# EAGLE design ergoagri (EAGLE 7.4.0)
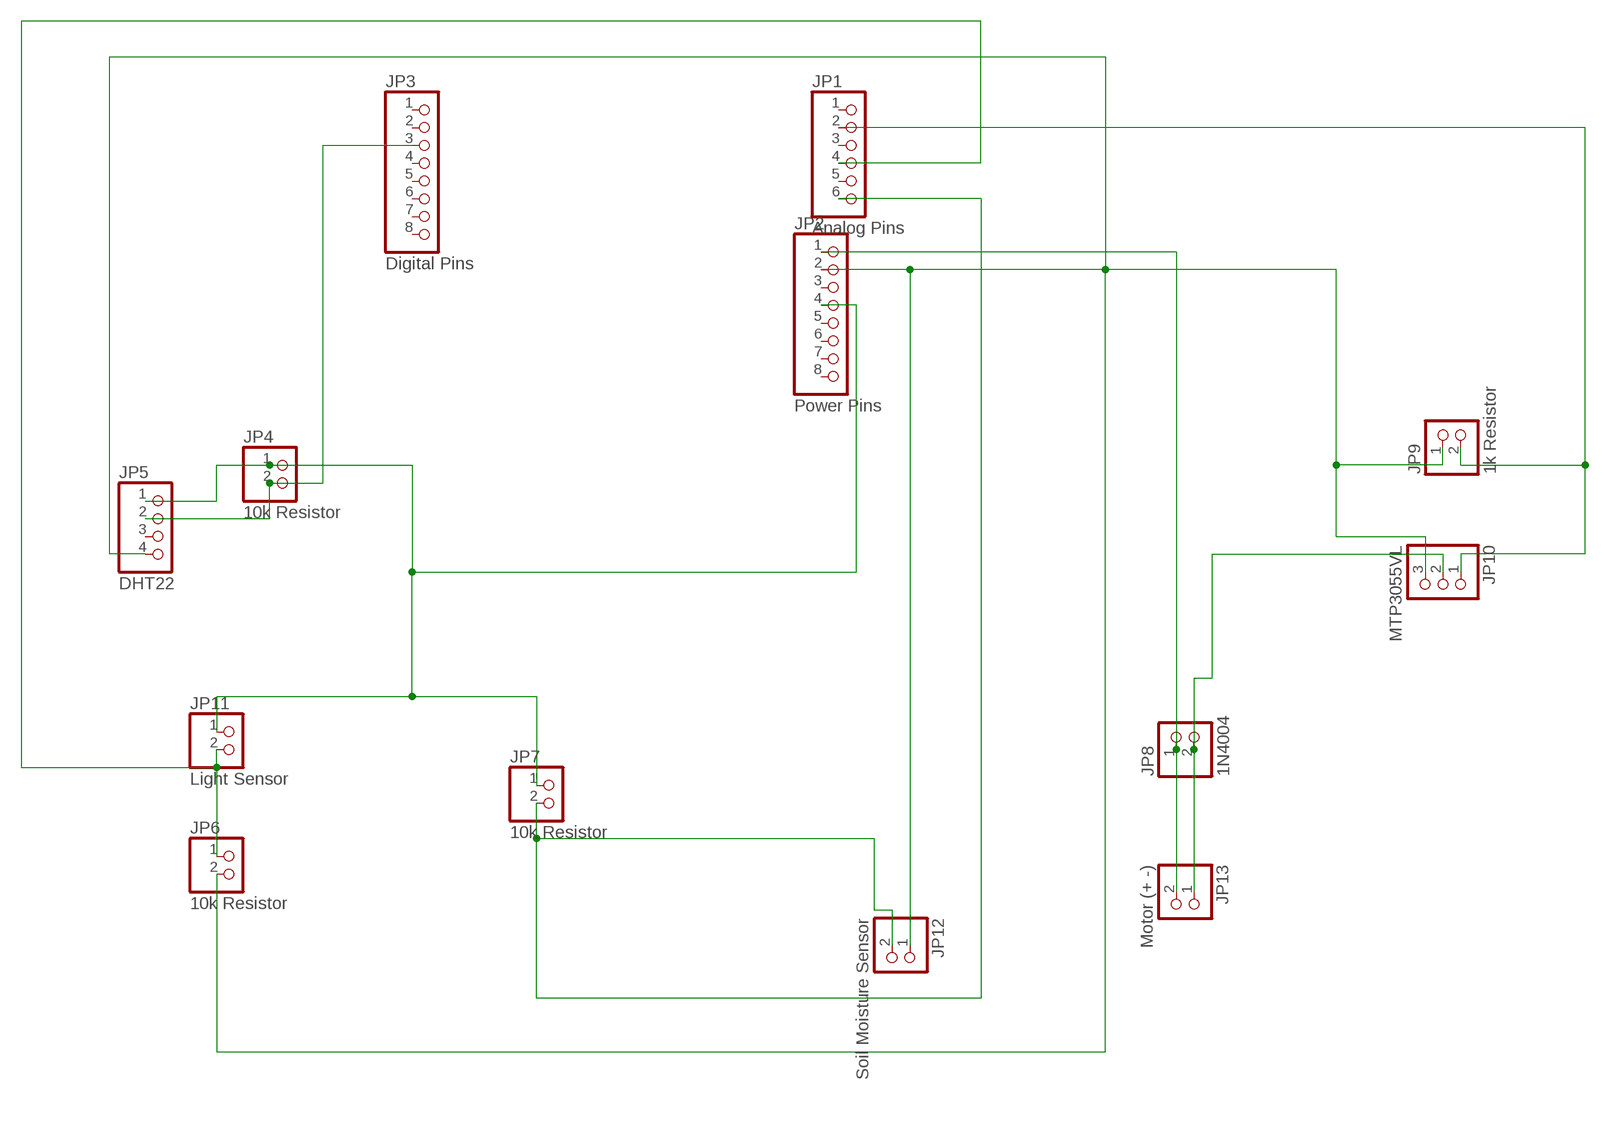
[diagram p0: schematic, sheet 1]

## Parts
JP1  Analog Pins  PINHD-1X6  [1X06]
JP2  Power Pins  PINHD-1X8  [1X08]
JP3  Digital Pins  PINHD-1X8  [1X08]
JP4  10k Resistor  PINHD-1X2  [1X02]
JP5  DHT22  PINHD-1X4  [1X04]
JP6  10k Resistor  PINHD-1X2  [1X02]
JP7  10k Resistor  PINHD-1X2  [1X02]
JP8  1N4004  PINHD-1X2  [1X02]
JP9  1k Resistor  PINHD-1X2  [1X02]
JP10  MTP3055VL  PINHD-1X3  [1X03]
JP11  Light Sensor  PINHD-1X2  [1X02]
JP12  Soil Moisture Sensor  PINHD-1X2  [1X02]
JP13  Motor (+ -)  PINHD-1X2  [1X02]

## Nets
B$2: JP1.6 JP7.2 JP12.2
N$2: JP8.2 JP10.2 JP13.1
N$3: JP2.4 JP4.1 JP5.1 JP7.1 JP11.1
N$4: JP3.3 JP4.2 JP5.2
N$5: JP1.2 JP9.2 JP10.1
N$6: JP2.2 JP5.4 JP6.2 JP9.1 JP10.3 JP12.1
N$7: JP2.1 JP8.1 JP13.2
N$9: JP1.4 JP6.1 JP11.2
Unconnected: JP1.1 JP1.3 JP1.5 JP2.3 JP2.5 JP2.6 JP2.7 JP2.8 JP3.1 JP3.2 JP3.4 JP3.5 JP3.6 JP3.7 JP3.8 JP5.3

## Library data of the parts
JP1 = pinhead:PINHD-1X6: PIN HEADER
JP2 JP3 = pinhead:PINHD-1X8: PIN HEADER
JP4 JP6-JP9 JP11-JP13 = pinhead:PINHD-1X2: PIN HEADER
JP5 = pinhead:PINHD-1X4: PIN HEADER
JP10 = pinhead:PINHD-1X3: PIN HEADER

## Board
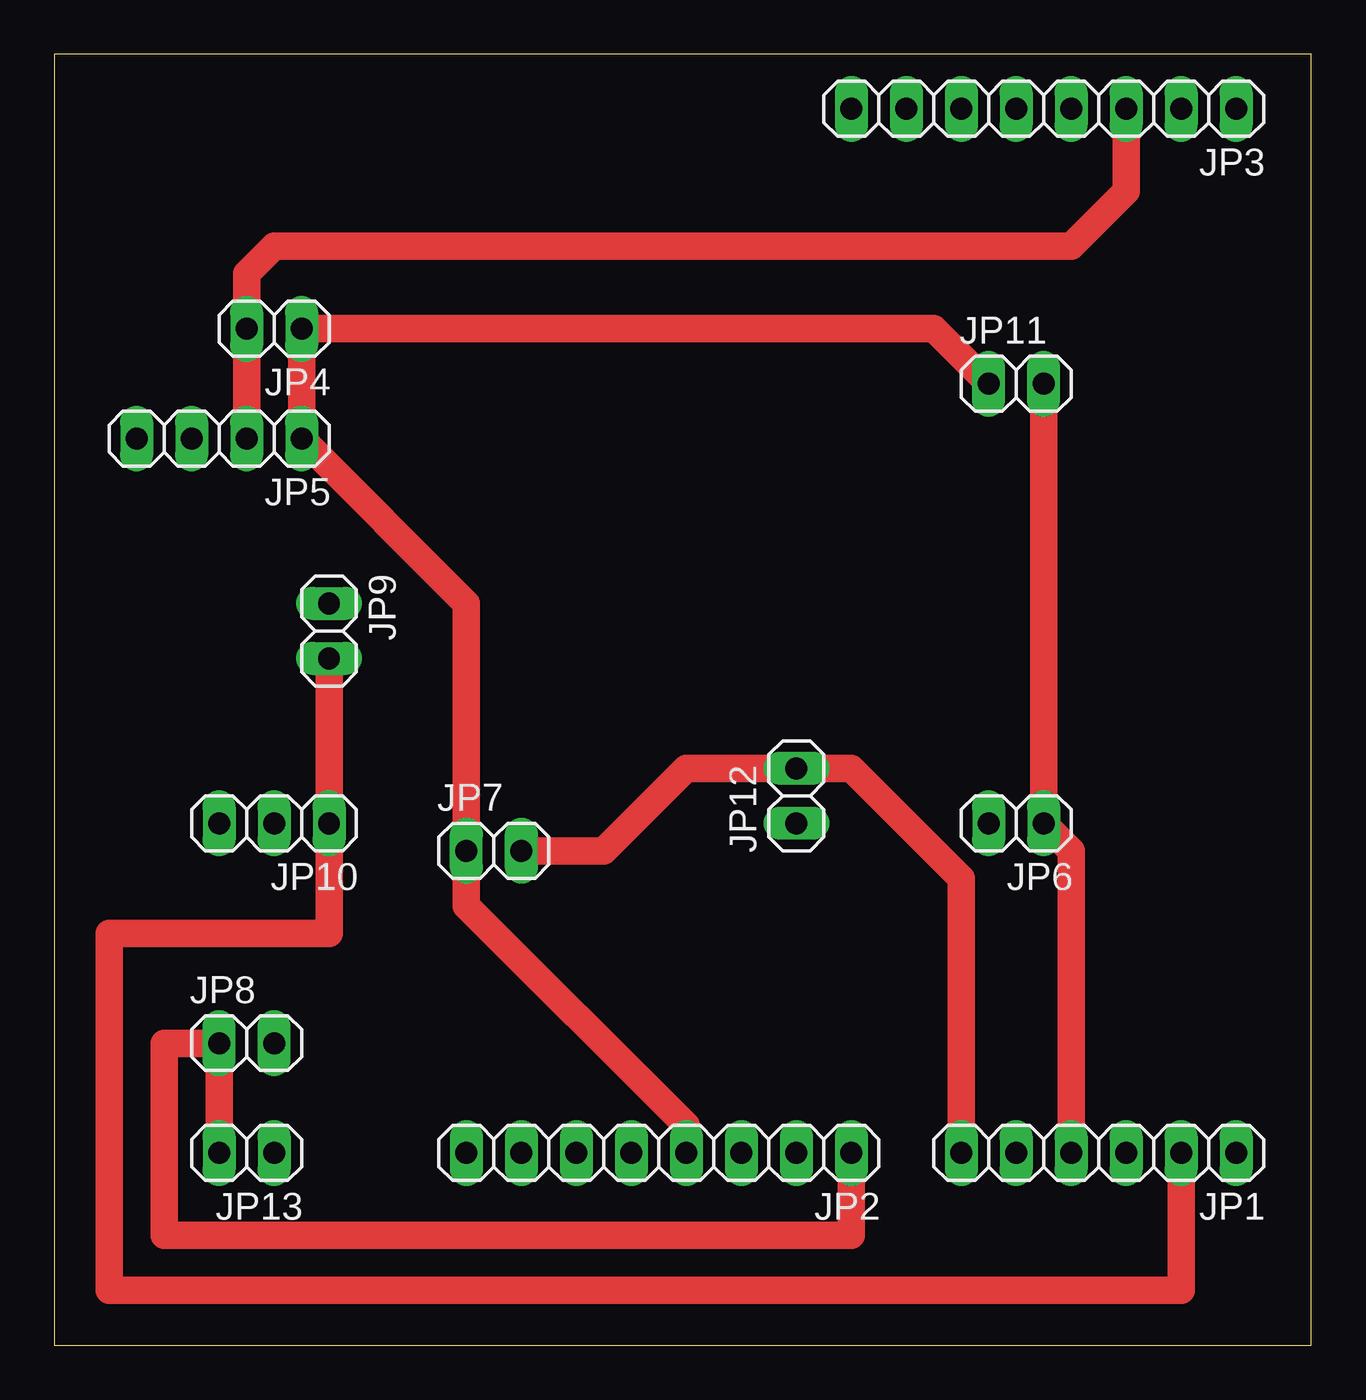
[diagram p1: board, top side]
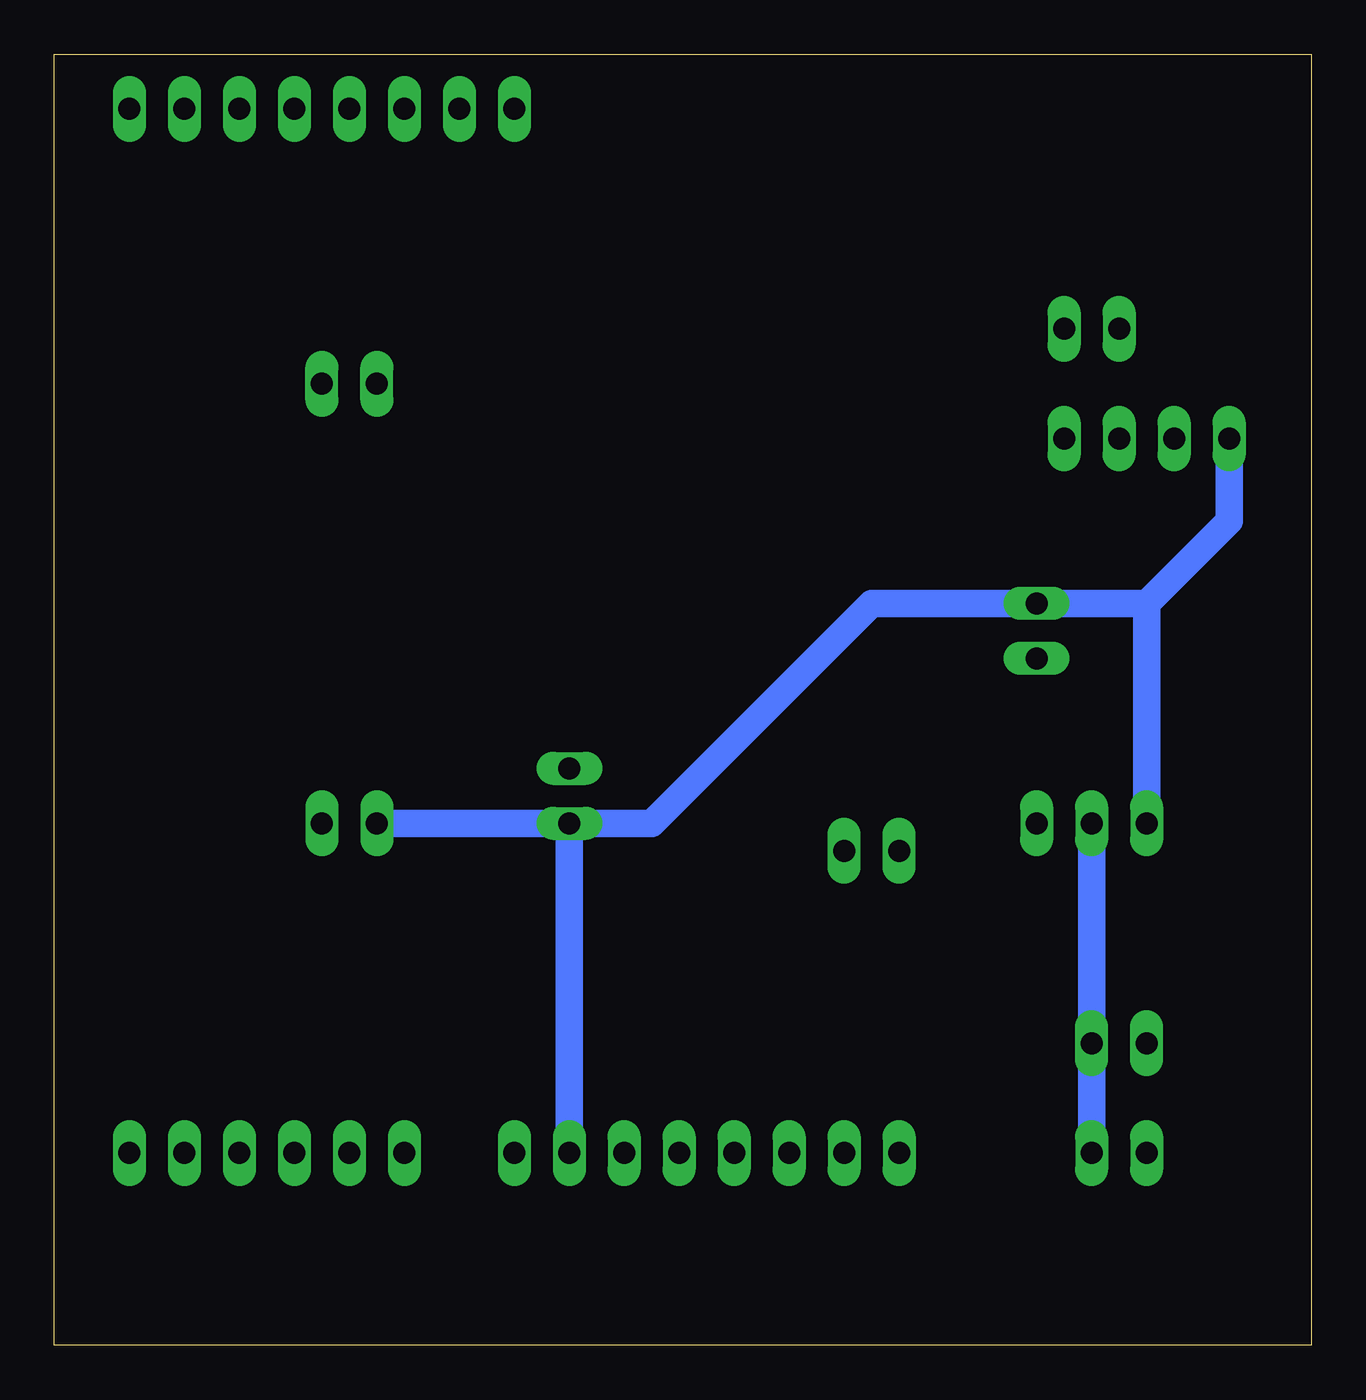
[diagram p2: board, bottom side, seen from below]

Size 58.09 x 59.68 mm. Coordinates in mm from the lower left corner, seen from the top.
Outline: 0,0 58.09,0 58.09,59.68 0,59.68 0,0
Copper layers (1*16): Top 0.035mm / dielectric 1.5mm / Bottom 0.035mm
Design rules "default": minimum track width 10mil, minimum drill 24mil, track to track 8mil, track to pad 8mil, pad to pad 8mil, via to via 8mil, smd to smd 8mil, copper to edge 40mil, drill to drill 8mil, minimum pad ring 10mil, minimum via ring 8mil, stop-mask expansion 4mil, vias tented up to drill 0mil, thermal gap 10mil

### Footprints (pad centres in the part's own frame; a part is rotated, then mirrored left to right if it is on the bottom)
1X06 = drill 1.016 long: 1 -6.35,0; 2 -3.81,0; 3 -1.27,0; 4 1.27,0; 5 3.81,0; 6 6.35,0
1X08 = drill 1.016 long: 1 -8.89,0; 2 -6.35,0; 3 -3.81,0; 4 -1.27,0; 5 1.27,0; 6 3.81,0; 7 6.35,0; 8 8.89,0
1X02 = drill 1.016 long: 1 -1.27,0; 2 1.27,0
1X04 = drill 1.016 long: 1 -3.81,0; 2 -1.27,0; 3 1.27,0; 4 3.81,0
1X03 = drill 1.016 long: 1 -2.54,0; 2 0,0; 3 2.54,0

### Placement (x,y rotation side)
JP1  48.26,8.89 180 top
JP2  27.94,8.89 180 top
JP3  45.72,57.15 180 top
JP4  10.16,46.99 180 top
JP5  7.62,41.91 180 top
JP6  44.45,24.13 180 top
JP7  20.32,22.86 0 top
JP8  8.89,13.97 0 top
JP9  12.7,33.02 270 top
JP10  10.16,24.13 180 top
JP11  44.45,44.45 0 top
JP12  34.29,25.4 90 top
JP13  8.89,8.89 180 top

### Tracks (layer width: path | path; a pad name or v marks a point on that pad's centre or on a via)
B$2
  Top 1.27: JP7.2 25.4,22.86 29.21,26.67 JP12.2 36.83,26.67 41.91,21.59 JP1.6
N$2
  Bottom 1.27: JP13.1 JP8.2 JP10.2
N$3
  Top 1.27: JP11.1 40.64,46.99 JP4.1 JP5.1 19.05,34.29 JP7.1 19.05,20.32 29.21,10.16 JP2.4
N$4
  Top 1.27: JP5.2 JP4.2 8.89,49.53 10.16,50.8 46.99,50.8 49.53,53.34 JP3.3
N$5
  Top 1.27: JP9.2 JP10.1 12.7,19.05 2.54,19.05 2.54,2.54 52.07,2.54 JP1.2
N$6
  Bottom 1.27: 7.62,34.29 JP9.1 20.32,34.29 30.48,24.13 JP12.1 | 7.62,34.29 JP10.3 | JP5.4 3.81,38.1 7.62,34.29 | JP12.1 JP6.2 | JP12.1 JP2.2
N$7
  Top 1.27: JP13.2 JP8.1 5.08,13.97 5.08,5.08 36.83,5.08 JP2.1
N$9
  Top 1.27: JP11.2 JP6.1 46.99,22.86 JP1.4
